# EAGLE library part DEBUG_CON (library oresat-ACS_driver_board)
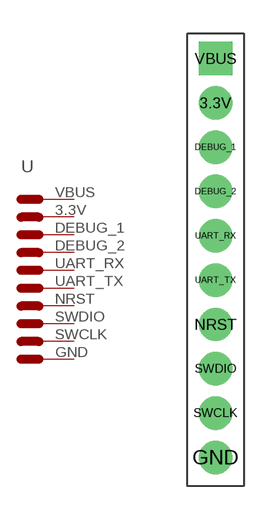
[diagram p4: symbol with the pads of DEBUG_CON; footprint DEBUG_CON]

Designator prefix -

## DEBUG_CON  [DEBUG_CON]
3.3V  2
DEBUG_1  3
DEBUG_2  4
GND  10
NRST  7
SWCLK  9
SWDIO  8
UART_RX  5
UART_TX  6
VBUS  1

## Footprint DEBUG_CON (pad centres in mm)
drill 1: 3.3V 0,6; DEBUG_1 0,4; DEBUG_2 0,2; GND 0,-10; NRST 0,-4; SWCLK 0,-8; SWDIO 0,-6; UART_RX 0,0; UART_TX 0,-2
drill 1 square: VBUS 0,8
